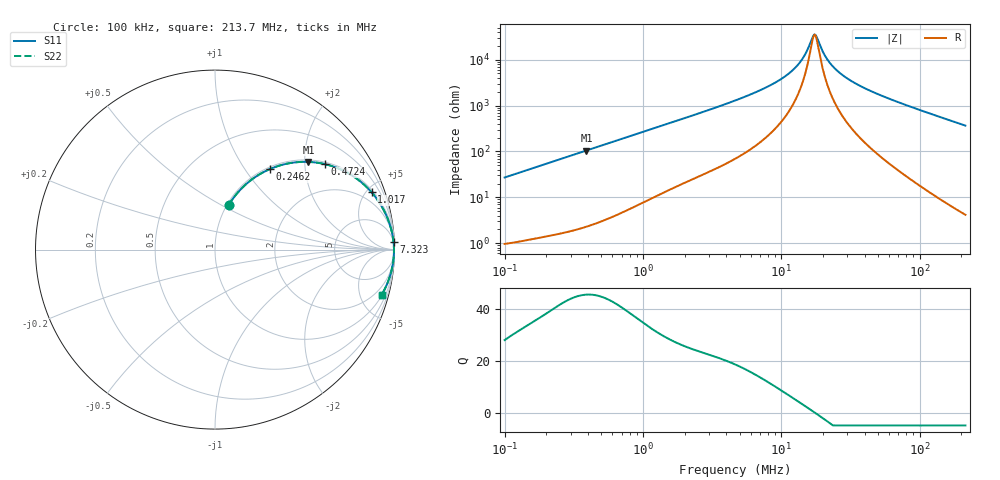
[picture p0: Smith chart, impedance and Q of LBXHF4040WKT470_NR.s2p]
! LBXHF4040WKT470_NR  S-PARAMETER MODEL  ( General Type )
! Model Generated by TAIYO YUDEN Corporation (http://www.ty-top.com)
! Version 1.0
! TAIYO YUDEN Control No. 210719NI43SB-FBB
! Copyright(c) 2021 TAIYO YUDEN CO.,LTD. All Rights Reserved.
! Product Description (link to TY-COMPAS)
! https://ds.yuden.co.jp/TYCOMPAS/or/detail?pn=LBXHF4040WKT470MNR&u=M
! Products Name : Inductors
! Characteristics :
!  Inductance : 47 uH , SRF(min) : 11 MHz , DC Resistance(max) : 0.66 Ohm
!  Rated Current : Saturation :700 mA , Temp Rise : 530 mA
!  Case Size : 4.0 x 4.0 / 0.157 x 0.157 [mm/inch] , Thickness : 2 / 0.079 [mm/inch]
!  (Conditions: Temperature = 25 degC , DC Bias Current/Voltage = 0A / 0V)
! External Node Assignments :
!  1  o---GGG---o  2
! GND o---------o GND
! Frequency Range : 0.1MHz  -  213.673535MHz  [ 402 STEP ]
# MHz S RI R 50
! Freq[MHz].  S11 Real  S11 Imag  S21 Real  S21 Imag  S12 Real  S12 Imag  S22 Real  S22 Imag
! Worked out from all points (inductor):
!   401 points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, 100 kHz to 213.7 MHz, reference 50 ohm
!   read as one part in series: L = 42.9 uH near 103.9 kHz
!   highest Q = 45.6 at 390 kHz (marker M1), where L = 42.6 uH
!   self-resonance near 17.35 MHz
!   S11 on the Smith chart (normalised r, x): 100 kHz: 1.02, +0.54; 246.2 kHz: 1.03, +1.32; 472.4 kHz: 1.06, +2.53; 1.017 MHz: 1.16, +5.41; 7.323 MHz: 4, +45; 213.7 MHz: 1.08, -7.31
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0.1  0.0758 0.2474  0.9242 -0.2474  0.9242 -0.2474  0.0758 0.2474
0.158411  0.1611 0.3535  0.8389 -0.3535  0.8389 -0.3535  0.1611 0.3535
0.246176  0.308 0.4498  0.692 -0.4498  0.692 -0.4498  0.308 0.4498
0.361188  0.4836 0.4888  0.5164 -0.4888  0.5164 -0.4888  0.4836 0.4888
0.38997  0.5209 0.4887  0.4791 -0.4887  0.4791 -0.4887  0.5209 0.4887
0.472362  0.6123 0.4763  0.3877 -0.4763  0.3877 -0.4763  0.6123 0.4763
0.693046  0.7684 0.4098  0.2316 -0.4098  0.2316 -0.4098  0.7684 0.4098
1.016833  0.8729 0.3188  0.1271 -0.3188  0.1271 -0.3188  0.8729 0.3188
1.304567  0.916 0.2615  0.084 -0.2615  0.084 -0.2615  0.916 0.2615
4.71194  0.9902 0.0751  0.00983 -0.0751  0.00983 -0.0751  0.9902 0.0751
7.322517  0.9948 0.0433  0.00524 -0.0433  0.00524 -0.0433  0.9948 0.0433
9.950627  0.9962 0.0262  0.00375 -0.0262  0.00375 -0.0262  0.9962 0.0262
12.524  0.9968 0.0149  0.00315 -0.0149  0.00315 -0.0149  0.9968 0.0149
14.5995  0.9971 0.00786  0.00293 -0.00786  0.00293 -0.00786  0.9971 0.00786
16.69585  0.9972 0.00184  0.00283 -0.00184  0.00283 -0.00184  0.9972 0.00184
17.68405  0.9972 -0.000727  0.00282 0.000727  0.00282 0.000727  0.9972 -0.000727
21.4203  0.9971 -0.00934  0.00287 0.00934  0.00287 0.00934  0.9971 -0.00934
23.57477  0.997 -0.0138  0.00296 0.0138  0.00296 0.0138  0.997 -0.0138
26.95988  0.9968 -0.0202  0.00316 0.0202  0.00316 0.0202  0.9968 -0.0202
37.345  0.9959 -0.0374  0.00414 0.0374  0.00414 0.0374  0.9959 -0.0374
60.30341  0.9922 -0.0705  0.00775 0.0705  0.00775 0.0705  0.9922 -0.0705
213.6735  0.9278 -0.2532  0.0722 0.2532  0.0722 0.2532  0.9278 -0.2532
